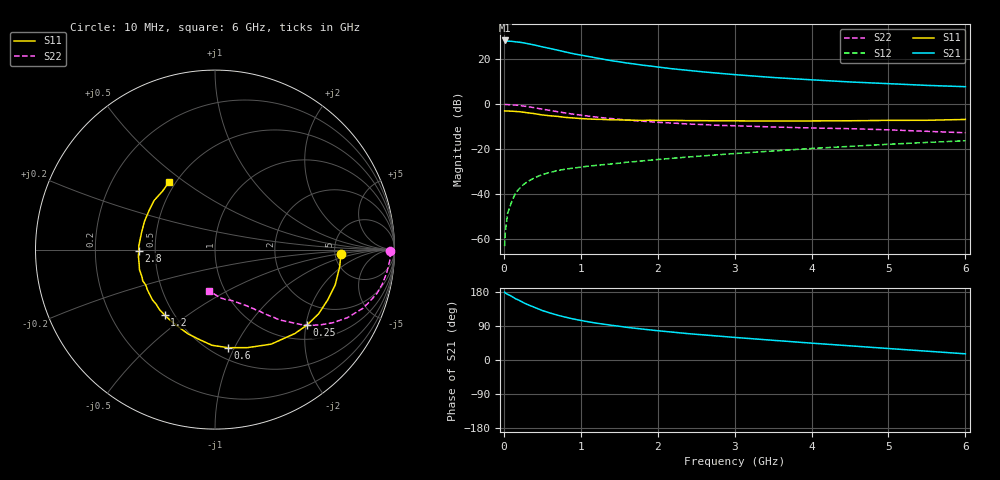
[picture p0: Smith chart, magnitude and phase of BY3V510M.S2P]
! SIEMENS Small Signal Semiconductors
! BFY420
! Si NPN RF SIEGET Grounded Emitter Transistor in MICRO-X
! VCE = 3.5 V  IC = 10 mA
! Common Emitter S-Parameters:  October  1996
# GHz  S  MA  R  50
!  f  S11  S21  S12  S22
! GHz  MAG  ANG  MAG  ANG  MAG  ANG  MAG  ANG
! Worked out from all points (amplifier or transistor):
!   36 points, 10 MHz to 6 GHz, reference 50 ohm
!   highest |S21| = 28.3 dB at 10 MHz (marker M1)
!   |S21| within 3 dB of that: start of sweep to 522.2 MHz
!   unconditionally stable (mu >= 1): 2.545 GHz to end of sweep
!   at 250 MHz: K = 0.21, MSG = 31.6 dB, |S12| = -35.9 dB
!   at 1.4 GHz: K = 0.75, MSG = 22.9 dB, |S12| = -26.6 dB
!   at 6 GHz: K = 1.09, MAG = 10.2 dB, |S12| = -16.3 dB
!   S11 on the Smith chart (normalised r, x): 10 MHz: 5.71, -0.50; 250 MHz: 1.35, -2.03; 600 MHz: 0.60, -0.94; 1.2 GHz: 0.44, -0.41; 2.8 GHz: 0.40, -0.01; 6 GHz: 0.46, +0.44
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0.01  0.7039 -1.8  25.93 178.9  0.0007 69.7  0.9764 -0.6
0.02  0.7012 -3.2  25.67 176.5  0.0015 67.3  0.978 -1.4
0.05  0.7012 -7.9  25.02 173.2  0.0038 74.9  0.9754 -3.8
0.1  0.698 -16.3  24.84 168.3  0.0066 78.4  0.9651 -7.8
0.15  0.6876 -24.1  24.2 161.9  0.0105 73.0  0.952 -11.6
0.2  0.6792 -31.8  23.74 157.4  0.0132 73.8  0.935 -15.1
0.25  0.6629 -39.4  23.03 151.8  0.0161 70.1  0.9088 -18.6
0.3  0.6453 -46.5  22.18 147.0  0.0186 68.4  0.8859 -21.7
0.4  0.6127 -59.3  20.52 138.9  0.0232 64.1  0.8293 -27.2
0.5  0.5753 -71.7  18.7 130.5  0.0272 60.0  0.7745 -31.7
0.6  0.5513 -82.5  17.21 124.1  0.0304 57.6  0.7231 -35.4
0.8  0.5072 -100.5  14.39 113.1  0.0359 52.7  0.6351 -41.1
0.9  0.4928 -107.7  13.2 108.4  0.0379 52.2  0.5992 -43.0
1.1  0.4674 -121.6  11.43 100.8  0.042 51.0  0.541 -46.8
1.2  0.4599 -127.6  10.62 97.3  0.0436 50.5  0.5157 -48.3
1.6  0.4411 -145.9  8.181 86.2  0.0513 49.5  0.4425 -52.9
2.2  0.4355 -165.0  6.071 73.4  0.0629 48.9  0.3792 -58.5
2.8  0.4253 -179.3  4.837 62.9  0.0753 47.7  0.3369 -63.5
3.5  0.4201 166.7  3.901 52.0  0.0911 45.1  0.3105 -68.9
4.5  0.427 149.4  3.106 37.4  0.1153 39.2  0.2849 -77.9
5.5  0.4375 131.9  2.607 23.3  0.1409 31.7  0.2487 -90.5
6  0.4564 123.9  2.437 16.3  0.1536 27.7  0.2311 -98.4
